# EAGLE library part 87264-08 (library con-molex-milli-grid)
RECEPTACAL
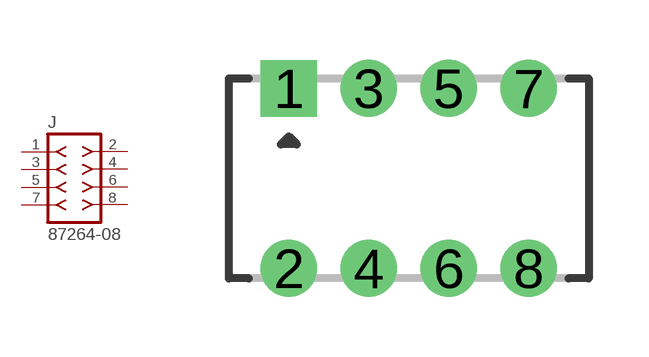
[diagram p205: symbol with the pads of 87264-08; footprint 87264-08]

Designator prefix J

## 87264-08  [87264-08]
1  1  pas
2  2  pas
3  3  pas
4  4  pas
5  5  pas
6  6  pas
7  7  pas
8  8  pas

## Footprint 87264-08 (pad centres in mm)
RECEPTACAL Dual Row, Side Entry
drill 0.914 square: 1 -3,2.25
drill 0.914: 2 -3,-2.25; 3 -1,2.25; 4 -1,-2.25; 5 1,2.25; 6 1,-2.25; 7 3,2.25; 8 3,-2.25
